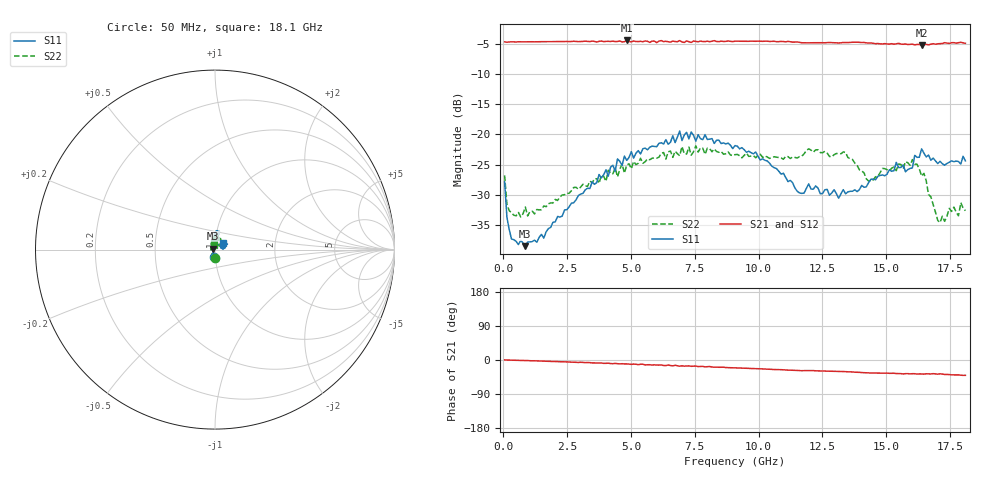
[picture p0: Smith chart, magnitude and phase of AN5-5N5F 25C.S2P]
! Network Analyzer HP8720D.06.14 Serial No. US36140669
!  5 Jul 2005  07:43:52
! Frequency  S11  S21  S12  S22
# HZ  S  DB R 50
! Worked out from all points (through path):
!   201 points, 50 MHz to 18.1 GHz, reference 50 ohm
!   highest |S21| = -4.45 dB at 4.833 GHz (marker M1); lowest = -5.2 dB at 16.39 GHz (marker M2)
!   group delay of S21, straight-line fit = 6.43 ps
!   lowest |S11| = -38.5 dB at 862.2 MHz (marker M3), VSWR 1.02, Z = 49 + j0.583 ohm
!   |S11| at or under -10 dB: start of sweep to end of sweep
!   |S22| runs from -34.6 to -21.9 dB; largest |S21 - S12| = 0.017
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5e7  -27.81 -101.5  -4.69 0.2  -4.70 0.5  -26.75 -92.3
1.4025e8  -33.69 -124.4  -4.74 -0.1  -4.72 0.0  -31.56 -138.2
3.2075e8  -37.30 -156.1  -4.67 -0.3  -4.70 -0.2  -32.92 -165.2
8.6225e8  -38.47 150.0  -4.68 -1.5  -4.69 -1.4  -32.00 167.0
1.22325e9  -37.48 135.7  -4.68 -2.2  -4.68 -2.2  -33.14 150.7
3.1185e9  -29.74 84.8  -4.61 -6.3  -4.64 -6.5  -28.23 122.4
4.83325e9  -24.28 81.6  -4.45 -10.3  -4.54 -10.9  -25.06 98.5
6.09675e9  -21.46 78.0  -4.57 -13.5  -4.51 -13.4  -23.75 91.8
6.909e9  -19.42 83.1  -4.47 -16.3  -4.57 -15.4  -23.53 81.7
9.075e9  -21.84 91.0  -4.57 -20.6  -4.56 -20.6  -23.34 71.0
1.1602e10  -29.66 93.5  -4.77 -27.9  -4.74 -28.1  -23.66 77.8
1.21435e10  -29.05 84.2  -4.83 -28.0  -4.79 -28.2  -22.93 77.5
1.313625e10  -30.54 57.3  -4.87 -30.2  -4.83 -30.6  -23.13 83.2
1.43095e10  -27.96 8.3  -4.88 -34.1  -4.85 -34.4  -27.72 85.9
1.512175e10  -25.82 10.7  -5.05 -35.2  -4.95 -35.0  -26.03 89.8
1.602425e10  -25.54 25.7  -5.06 -36.2  -5.18 -37.4  -24.16 63.9
1.638525e10  -22.38 23.8  -5.25 -36.8  -5.09 -36.7  -26.89 47.5
1.710725e10  -24.44 25.9  -4.97 -36.5  -4.95 -37.0  -34.56 68.0
1.746825e10  -24.59 34.2  -4.94 -38.5  -4.93 -38.4  -32.22 89.7
1.782925e10  -24.47 39.1  -4.82 -39.4  -4.85 -39.2  -33.45 98.6
1.79195e10  -24.89 38.3  -4.75 -40.0  -4.66 -39.8  -31.27 104.2
1.81e10  -24.37 39.3  -4.93 -40.5  -4.95 -41.3  -32.60 99.6
